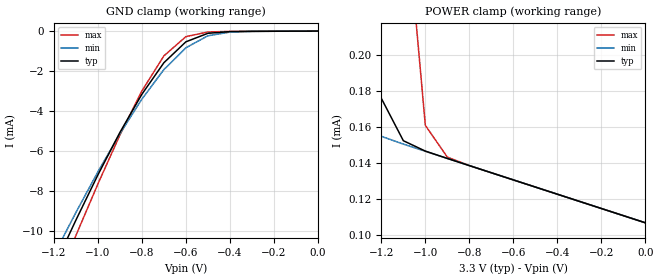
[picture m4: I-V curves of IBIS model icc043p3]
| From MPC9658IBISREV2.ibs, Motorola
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|This model is an Input with a 25,000 ohm Pull_down at 3.3V
[Model]   icc043p3
Model_type   Input
Vref=1.5V
Vinl=0.8V
Vinh=2.0V
| Variable   typ   min   max
C_comp   5p   5p   5p
[Temperature Range]   27.00   100.00   -45.00
[Power Clamp Reference]   3.30V   3.00V   3.60V
[Gnd Clamp Reference]   0.000V   0.000V   0.000V
[Voltage Range]   3.30V   3.00V   3.60V
[Pulldown Reference]   0.000V   0.000V   0.000V
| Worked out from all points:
|   GND clamp passes 1 mA (typ) near -0.64 V on its own axis
|   POWER clamp passes 1 mA (typ) near -1.44 V on its own axis
[GND_clamp]
| voltage   I(typ)   I(min)   I(max)
-3.3V     -65.45mA   -61.69mA   -70.25mA
-1.2V     -11.83mA   -11.21mA   -12.91mA
-1.1V     -9.467mA   -9.084mA   -10.24mA
-1V       -7.201mA   -7.048mA   -7.655mA
-900mV    -5.077mA   -5.139mA   -5.207mA
-800mV    -3.163mA   -3.405mA   -2.998mA
-700mV    -1.585mA   -1.928mA   -1.242mA
-600mV    -537uA     -834.6uA   -278.5uA
-500mV    -111.2uA   -235.5uA   -44.5uA
-400mV    -25.07uA   -49.72uA   -17.01uA
1.97fV    -61.68pA   -9.69nA    -3.014pA
[POWER_clamp]
| voltage   I(typ)  I(min)  I(max)
-3.3V     27.21mA    21.56mA    34.07mA
-1.5V     1.4mA      337.1uA    3.859mA
-1.4V     717.9uA    194.4uA    2.632mA
-1.3V     311.6uA    162.1uA    1.579mA
-1.2V     175.9uA    154.8uA    767.8uA
-1.1V     152.4uA    150.5uA    297.2uA
-1V       146.6uA    146.5uA    160.9uA
-900mV    142.6uA    142.6uA    143.3uA
-800mV    138.6uA    138.6uA    138.6uA
1.97fV    106.9uA    106.9uA    106.9uA
